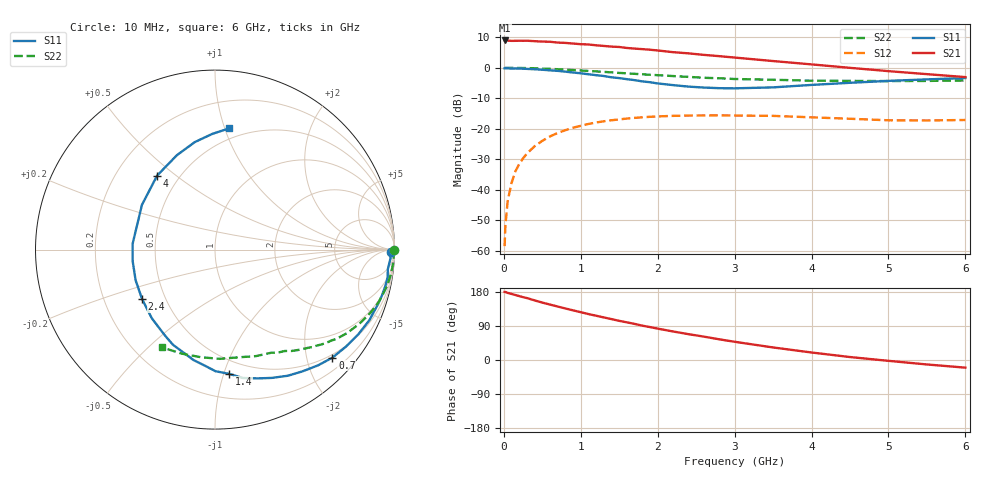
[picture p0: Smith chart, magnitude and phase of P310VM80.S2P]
! SIEMENS Small Signal Semiconductors
! BFP181
! Si NPN RF Bipolar Junction Transistor in SOT143
! VCE = 10 V  IC = 0.8 mA
! Common Emitter S-Parameters:  March  1996
# GHz  S  MA  R  50
!  f  S11  S21  S12  S22
! GHz  MAG  ANG  MAG  ANG  MAG  ANG  MAG  ANG
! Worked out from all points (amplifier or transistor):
!   36 points, 10 MHz to 6 GHz, reference 50 ohm
!   highest |S21| = 8.9 dB at 10 MHz (marker M1)
!   |S21| within 3 dB of that: start of sweep to 1.882 GHz
!   unconditionally stable (mu >= 1): 3.52 GHz to end of sweep
!   at 250 MHz: K = 0.09, MSG = 19.2 dB, |S12| = -29.7 dB
!   at 1.4 GHz: K = 0.45, MSG = 12.1 dB, |S12| = -17.2 dB
!   at 6 GHz: K = 1.33, MAG = 3.6 dB, |S12| = -17.1 dB
!   S11 on the Smith chart (normalised r, x): 10 MHz: 69, -38; 700 MHz: 0.44, -2.50; 1.4 GHz: 0.39, -1.04; 2.4 GHz: 0.37, -0.27; 4 GHz: 0.38, +0.43; 6 GHz: 0.41, +1.03
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0.01  0.978 -0.7  2.798 179.6  0.0012 80.4  0.9977 -0.2
0.02  0.977 -1.1  2.785 179.5  0.0026 93.0  0.994 -0.5
0.05  0.9792 -2.8  2.781 177.1  0.0066 92.1  0.9957 -1.5
0.1  0.9693 -6.4  2.755 174.4  0.013 85.4  0.9957 -2.9
0.15  0.9742 -9.2  2.759 171.5  0.0201 82.7  0.9946 -4.4
0.3  0.9577 -18.5  2.77 163.5  0.0394 77.4  0.9869 -8.9
0.4  0.9457 -24.6  2.724 157.3  0.0519 73.3  0.9805 -11.8
0.6  0.9076 -36.7  2.662 146.3  0.0752 65.0  0.9587 -17.5
0.7  0.889 -42.6  2.583 141.1  0.0855 61.1  0.9453 -20.2
0.8  0.8636 -48.3  2.551 136.0  0.0951 57.1  0.9315 -22.6
1.1  0.7819 -66.1  2.404 121.2  0.1202 46.7  0.8863 -29.7
1.4  0.6972 -83.4  2.22 107.9  0.1382 37.4  0.84 -36.3
1.5  0.6774 -89.8  2.188 103.3  0.1427 34.6  0.8229 -38.0
1.8  0.5981 -107.5  2.018 90.6  0.1544 27.5  0.7814 -43.1
2.2  0.5199 -132.6  1.798 75.3  0.1631 18.5  0.7312 -49.7
2.4  0.4911 -145.8  1.721 68.2  0.165 14.6  0.7088 -52.8
3  0.4603 176.1  1.469 48.1  0.165 5.1  0.6544 -61.4
3.5  0.4773 148.5  1.287 33.1  0.163 -0.9  0.6359 -68.9
4  0.5236 128.0  1.135 19.8  0.1543 -5.0  0.6143 -77.7
4.5  0.5672 112.0  0.997 7.8  0.1462 -8.0  0.6093 -87.5
5.5  0.645 91.3  0.786 -11.8  0.1371 -5.6  0.6087 -108.0
6  0.6792 83.5  0.703 -20.2  0.1396 -4.0  0.62 -118.7
